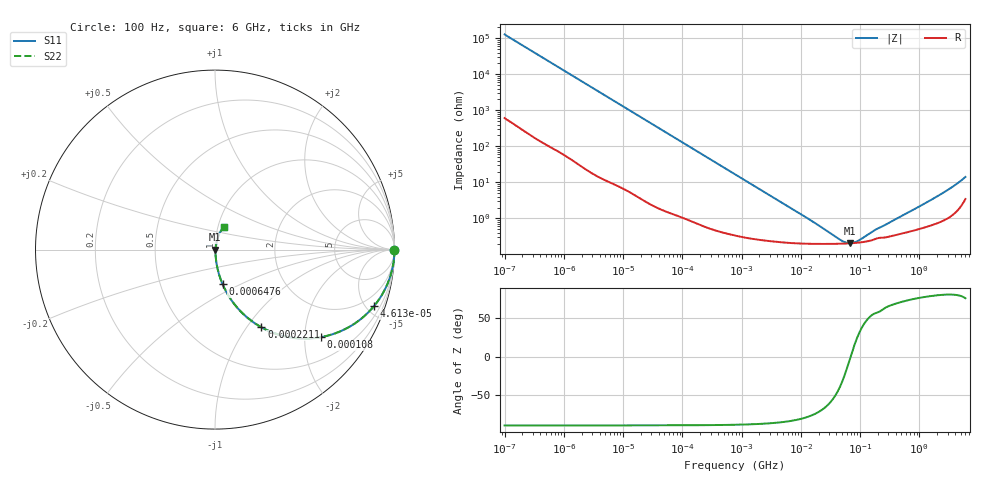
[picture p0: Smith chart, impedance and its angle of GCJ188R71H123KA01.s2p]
!Murata Part Number: GCJ188R71H123KA01
!These Parameters are Measured in Series Mode Connection
!Data Generated on Mar 13, 2026
!  o--ll--o
!Port1  Port2
!  o------o
!Operation Temp=25[degC], DC Bias Voltage=0[V]
!Freq. Start=100[Hz] Stop=6[GHz] 401[Steps]
# Hz S RI R 50
!Freq.(Hz) S11(Real) S11(Imag) S21(Real) S21(Imag) S12(Real) S12(Imag) S22(Real) S22(Imag)
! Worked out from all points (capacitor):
!   401 points, 100 Hz to 6 GHz, reference 50 ohm
!   read as one part in series: C = 12.5 nF near 109 Hz
!   lowest |Z| = 204 mohm at 68.17 MHz (marker M1)
!   series resonance near 69.46 MHz, so ESL is about 420 pH
!   S11 on the Smith chart (normalised r, x): 100 Hz: open; 46.13 kHz: 1.03, -5.59; 108 kHz: 1.02, -2.40; 221.1 kHz: 1.01, -1.18; 647.6 kHz: 1.01, -0.40; 6 GHz: 1.07, +0.27
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100  1 -0.000789  4.4e-06 0.000789  4.4e-06 0.000789  1 -0.000789
2008  0.9997 -0.0157  0.000313 0.0157  0.000313 0.0157  0.9997 -0.0157
12041  0.9908 -0.0928  0.00918 0.0928  0.00918 0.0928  0.9908 -0.0928
22537  0.9694 -0.1694  0.0306 0.1694  0.0306 0.1694  0.9694 -0.1694
40335  0.9096 -0.2839  0.0904 0.2839  0.0904 0.2839  0.9096 -0.2839
46134  0.8852 -0.3158  0.1148 0.3158  0.1148 0.3158  0.8852 -0.3158
69028  0.7764 -0.4132  0.2236 0.4132  0.2236 0.4132  0.7764 -0.4132
108014  0.5889 -0.4879  0.4111 0.4879  0.4111 0.4879  0.5889 -0.4879
154540  0.414 -0.4879  0.586 0.4879  0.586 0.4879  0.414 -0.4879
221108  0.2588 -0.4328  0.7412 0.4328  0.7412 0.4328  0.2588 -0.4328
361830  0.1178 -0.316  0.8822 0.316  0.8822 0.316  0.1178 -0.316
647581  0.0422 -0.1924  0.9578 0.1924  0.9578 0.1924  0.0422 -0.1924
774597  0.0307 -0.163  0.9693 0.163  0.9693 0.163  0.0307 -0.163
2481164  0.0052 -0.0526  0.9948 0.0526  0.9948 0.0526  0.0052 -0.0526
1.555665e7  0.00203 -0.00808  0.998 0.00808  0.998 0.00808  0.00203 -0.00808
4.764863e7  0.00198 -0.00146  0.998 0.00146  0.998 0.00146  0.00198 -0.00146
6.817316e7  0.00203 -6.99e-05  0.998 6.99e-05  0.998 6.99e-05  0.00203 -6.99e-05
9.326766e7  0.00212 0.00112  0.9979 -0.00112  0.9979 -0.00112  0.00212 0.00112
1.745687e8  0.00263 0.00384  0.9974 -0.00384  0.9974 -0.00384  0.00263 0.00384
3.124326e8  0.00317 0.00695  0.9968 -0.00695  0.9968 -0.00695  0.00317 0.00695
2.048624e9  0.00901 0.0404  0.991 -0.0404  0.991 -0.0404  0.00901 0.0404
6e9  0.05 0.1258  0.95 -0.1258  0.95 -0.1258  0.05 0.1258
